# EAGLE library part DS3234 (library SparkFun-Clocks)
Maxim DS3234 - Extremely Accurate SPI RTC The DS3234 is a low-cost, extremely accurate SPI™ bus real-time clock (RTC) with an integrated temperature-compensated crystal oscillator (TCXO) and crystal. SparkFun Products: Real Time Clock - DS3234 (COM-10079) SparkFun DeadOn RTC Breakout (BOB-10160) Datasheet
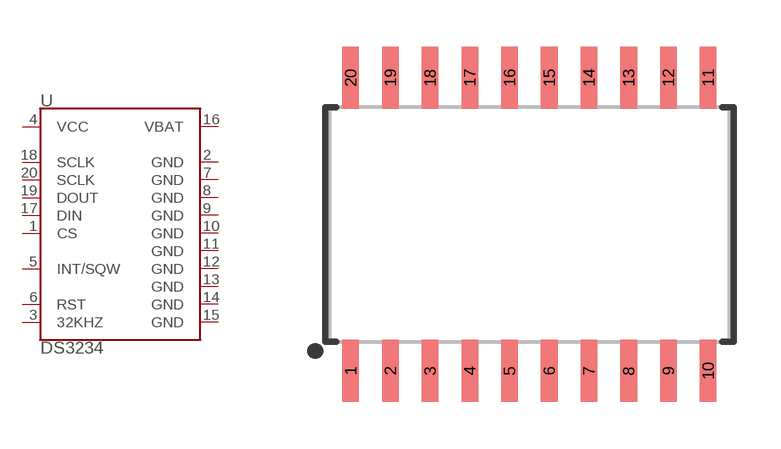
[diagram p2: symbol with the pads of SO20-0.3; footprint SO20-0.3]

Designator prefix U

## DS3234 (PROD_ID: IC-10016; SF_ID: COM-10079)  [SO20-0.3]
1  CS
2  GND
3  32KHZ
4  VCC
5  INT/SQW
6  RST
7  GND
8  GND
9  GND
10  GND
11  GND
12  GND
13  GND
14  GND
15  GND
16  VBAT
17  DIN
18  SCLK
19  DOUT
20  SCLK

## Footprint SO20-0.3 (pad centres in mm)
20-Pin SOIC (0.3" Wide) Dimensions: ~0.5x0.3" Package used by Maxim DS3234 SPI RTC Package Outline (W20#H2) Land Pattern
smd 0.53 x 1.98: 1 -5.715,-4.685; 2 -4.445,-4.685; 3 -3.175,-4.685; 4 -1.905,-4.685; 5 -0.635,-4.685; 6 0.635,-4.685; 7 1.905,-4.685; 8 3.175,-4.685; 9 4.445,-4.685; 10 5.715,-4.685; 11 5.715,4.685; 12 4.445,4.685; 13 3.175,4.685; 14 1.905,4.685; 15 0.635,4.685; 16 -0.635,4.685; 17 -1.905,4.685; 18 -3.175,4.685; 19 -4.445,4.685; 20 -5.715,4.685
